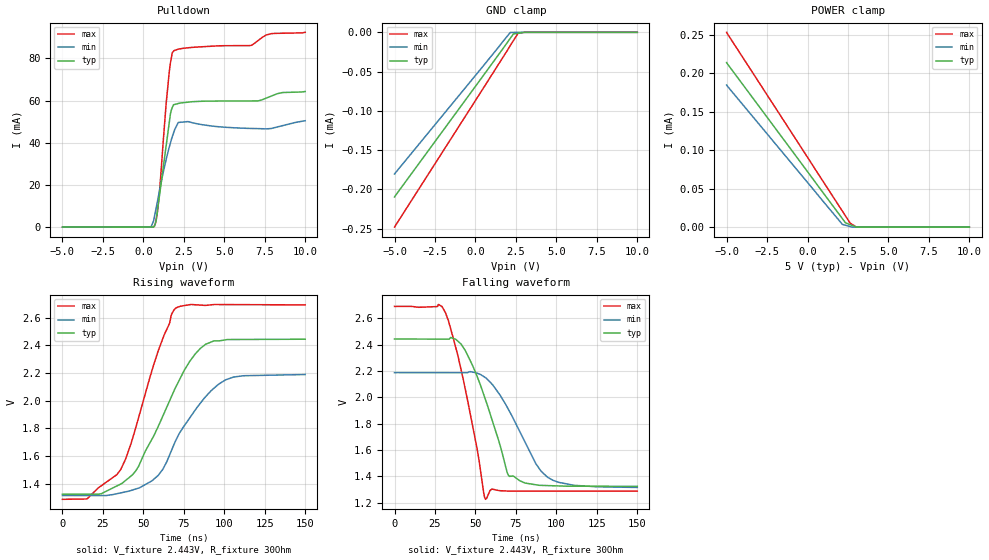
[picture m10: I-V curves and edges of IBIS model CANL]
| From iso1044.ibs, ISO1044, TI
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[Model]   CANL
Model_type   I/O_open_drain
Polarity   Non-Inverting
Enable   Active-Low
Vinl = 0.5
Vinh = 0.9
Vmeas = 2
Vref = 2.443
Cref = 2pF
Rref = 30
|   typ   min   max
C_comp   11.96e-12   11.44e-12   12.21e-12
[Voltage Range]   5   4.5   5.5
[Temperature Range]   25   150   -55
[Pullup Reference]   5   4.5   5.5
[Pulldown Reference]   0   0   0
[Power Clamp Reference]   5   4.5   5.5
[GND Clamp Reference]   0   0   0
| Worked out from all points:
|   slope of the pulldown table from 0 to 0.75 V, typ, clamps not added: 373 ohm
|   falling waveform, V_fixture 2.443V, R_fixture 30Ohm: 20-80 % time 18.1ns typ, 22.3ns min, 14.4ns max; typ from 2.44 V to 1.32 V
|   rising waveform, V_fixture 2.443V, R_fixture 30Ohm: 20-80 % time 27.4ns typ, 26.3ns min, 22.2ns max; typ from 1.32 V to 2.44 V
[Pulldown]
|   Voltage   I(typ)   I(min)   I(max)
-5V       30fA       -53.22pA   460fA
252.8mV   4.719uA    -3.121uA   -1.871uA
647.3mV   194.8uA    3.573mA    145.6uA
782.7mV   2.825mA    8.677mA    2.945mA
979mV     13.95mA    16.53mA    15.09mA
1.407V    38.49mA    32.05mA    58.45mA
1.6V      49.55mA    37.9mA     73.56mA
1.894V    58.11mA    45.29mA    83.7mA
2.755V    59.27mA    50.08mA    85.07mA
6.669V    59.86mA    46.81mA    86.22mA
7.601V    61.23mA    46.63mA    91.14mA
10V       64.34mA    50.49mA    92.41mA
[GND Clamp]
|   Voltage   I(typ)   I(min)   I(max)
-5V       -209.7uA   -180.5uA   -248.2uA
2.155V    -7.531uA   -153.4nA   -16.77uA
2.349V    -2.037uA   -103.9nA   -10.51uA
2.638V    -1.181uA   -29.97nA   -1.117uA
3.037V    0A         0A         0A
10V       0A         0A         0A
[POWER Clamp]
|   Voltage   I(typ)   I(min)   I(max)
-5V       213.6uA    184.5uA    252.9uA
2.155V    11.02uA    3.595uA    20.77uA
2.349V    5.558uA    2.436uA    14.52uA
2.638V    3.222uA    702.3nA    5.157uA
3.031V    53.18nA    0A         0A
10V       0A         0A         0A
[Ramp]
R_load = 30
|   typ   min   max
dV/dt_r   0.671493/2.72876e-08   0.524178/2.61335e-08   0.842197/2.20483e-08
dV/dt_f   0.671494/1.80697e-08   0.523421/2.22127e-08   0.842202/1.44627e-08
[Falling Waveform]
V_fixture = 2.443V
V_fixture_min = 2.188V
V_fixture_max = 2.691V
R_fixture = 30Ohm
C_fixture = 0F
|   Time   V(typ)   V(min)   V(max)
0s        2.443V     2.188V     2.691V
27.22ns   2.443V     2.188V     2.706V
31.4ns    2.443V     2.188V     2.646V
41.22ns   2.404V     2.188V     2.205V
56.2ns    1.983V     2.15V      1.226V
60.2ns    1.832V     2.101V     1.303V
71.01ns   1.4V       1.894V     1.288V
87.3ns    1.336V     1.497V     1.288V
94.67ns   1.33V      1.393V     1.288V
150ns     1.324V     1.316V     1.288V
[Rising Waveform]
V_fixture = 2.443V
V_fixture_min = 2.188V
V_fixture_max = 2.691V
R_fixture = 30Ohm
C_fixture = 0F
|   Time   V(typ)   V(min)   V(max)
0s        1.324V     1.315V     1.288V
15.16ns   1.324V     1.315V     1.29V
35.89ns   1.397V     1.334V     1.5V
45.28ns   1.493V     1.362V     1.803V
59.14ns   1.813V     1.46V      2.358V
67.49ns   2.033V     1.643V     2.626V
70ns      2.097V     1.711V     2.668V
85.22ns   2.377V     1.982V     2.69V
100.8ns   2.439V     2.15V      2.694V
150ns     2.444V     2.189V     2.691V
